(* Logix 5000 AddOnInstructionDefinition export Banner_QCM50_K3_K5_PD_v4; software revision 33.00 *)

TYPE Banner_QCM50_K3_K5_PDI_v4 :
STRUCT
   Signal_Quality : INT;   // 0 = no signal, 1 = overflow, 2 to 100.
   Switching_Quality : SINT;
   Q1 : SINT;
   Q2 : SINT;
   Q3 : SINT;
   Q4 : SINT;
   Q5 : SINT;
   Q6 : SINT;
   Q7 : SINT;
   Q8 : SINT;
   Q9 : SINT;
   Q10 : SINT;
   Q11 : SINT;
   Q12 : SINT;
   PDI_DT : SINT[6];
   Ratio_Red : INT;   // 0 = No Signal, 1 = Overflow, 10 to 4095 Ratio Value.
   Ratio_Green : INT;   // 0 = No Signal, 1 = Overflow, 10 to 4095 Ratio Value.
   Ratio_Blue : INT;   // 0 = No Signal, 1 = Overflow, 10 to 4095 Ratio Value.
   Energy : INT;   // 0 = No Signal, 1 = Overflow, 10 to 4095 Ratio Value.
END_STRUCT
END_TYPE

ADD_ON_INSTRUCTION Banner_QCM50_K3_K5_PD_v4   (* revision 4.0, vendor Banner Engineering *)
// Revision note:
// Updated Process data for correct addressing of Q1 through Q4.
VAR_IN_OUT
   PDI : Banner_QCM50_K3_K5_PDI_v4; {required}
END_VAR
VAR_INPUT
   Byte_Swap : BOOL; {required}
   K : DINT; {required}
   ProcessDataMapping : SINT; {required}
END_VAR
VAR
   Temp_Byte : SINT[6]; {access None}
END_VAR

ROUTINE Logic   (* ladder *)
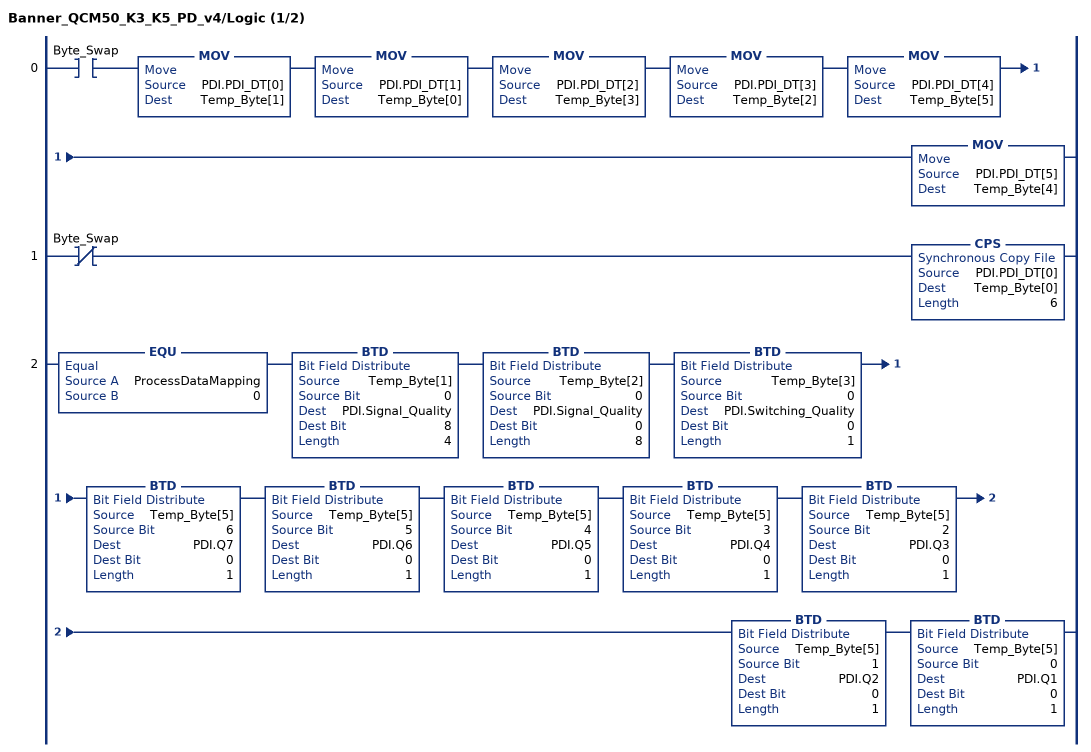
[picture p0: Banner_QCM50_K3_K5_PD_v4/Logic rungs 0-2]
   0: XIC(Byte_Swap)MOV(PDI.PDI_DT[0],Temp_Byte[1])MOV(PDI.PDI_DT[1],Temp_Byte[0])MOV(PDI.PDI_DT[2],Temp_Byte[3])MOV(PDI.PDI_DT[3],Temp_Byte[2])MOV(PDI.PDI_DT[4],Temp_Byte[5])MOV(PDI.PDI_DT[5],Temp_Byte[4]);
   1: XIO(Byte_Swap)CPS(PDI.PDI_DT[0],Temp_Byte[0],6);
   2: EQU(ProcessDataMapping,0)BTD(Temp_Byte[1],0,PDI.Signal_Quality,8,4)BTD(Temp_Byte[2],0,PDI.Signal_Quality,0,8)BTD(Temp_Byte[3],0,PDI.Switching_Quality,0,1)BTD(Temp_Byte[5],6,PDI.Q7,0,1)BTD(Temp_Byte[5],5,PDI.Q6,0,1)BTD(Temp_Byte[5],4,PDI.Q5,0,1)BTD(Temp_Byte[5],3,PDI.Q4,0,1)BTD(Temp_Byte[5],2,PDI.Q3,0,1)BTD(Temp_Byte[5],1,PDI.Q2,0,1)BTD(Temp_Byte[5],0,PDI.Q1,0,1);
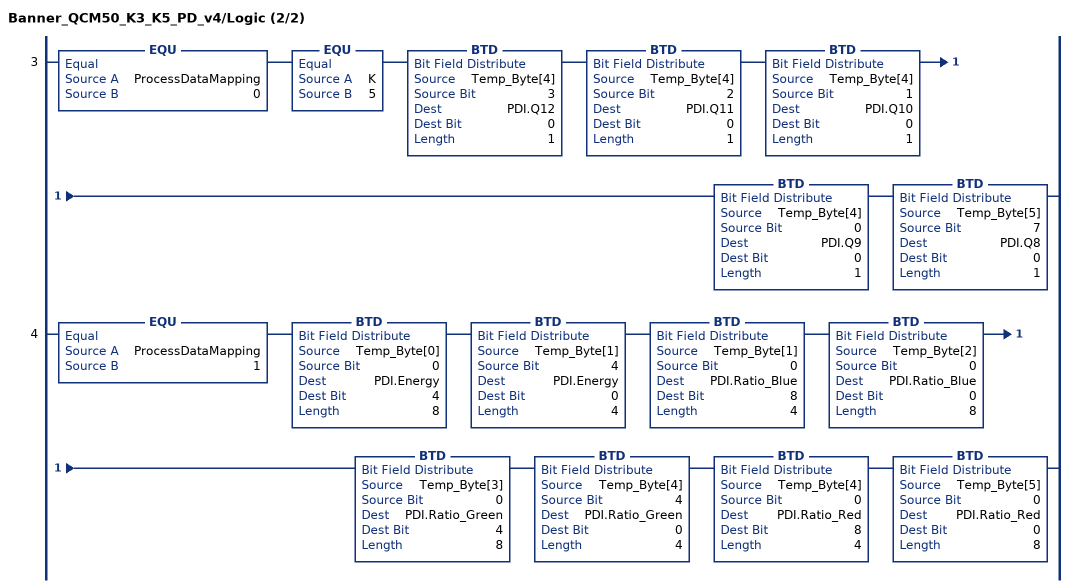
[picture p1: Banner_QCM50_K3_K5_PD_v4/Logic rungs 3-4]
   3: EQU(ProcessDataMapping,0)EQU(K,5)BTD(Temp_Byte[4],3,PDI.Q12,0,1)BTD(Temp_Byte[4],2,PDI.Q11,0,1)BTD(Temp_Byte[4],1,PDI.Q10,0,1)BTD(Temp_Byte[4],0,PDI.Q9,0,1)BTD(Temp_Byte[5],7,PDI.Q8,0,1);
   4: EQU(ProcessDataMapping,1)BTD(Temp_Byte[0],0,PDI.Energy,4,8)BTD(Temp_Byte[1],4,PDI.Energy,0,4)BTD(Temp_Byte[1],0,PDI.Ratio_Blue,8,4)BTD(Temp_Byte[2],0,PDI.Ratio_Blue,0,8)BTD(Temp_Byte[3],0,PDI.Ratio_Green,4,8)BTD(Temp_Byte[4],4,PDI.Ratio_Green,0,4)BTD(Temp_Byte[4],0,PDI.Ratio_Red,8,4)BTD(Temp_Byte[5],0,PDI.Ratio_Red,0,8);
END_ROUTINE
END_ADD_ON_INSTRUCTION
